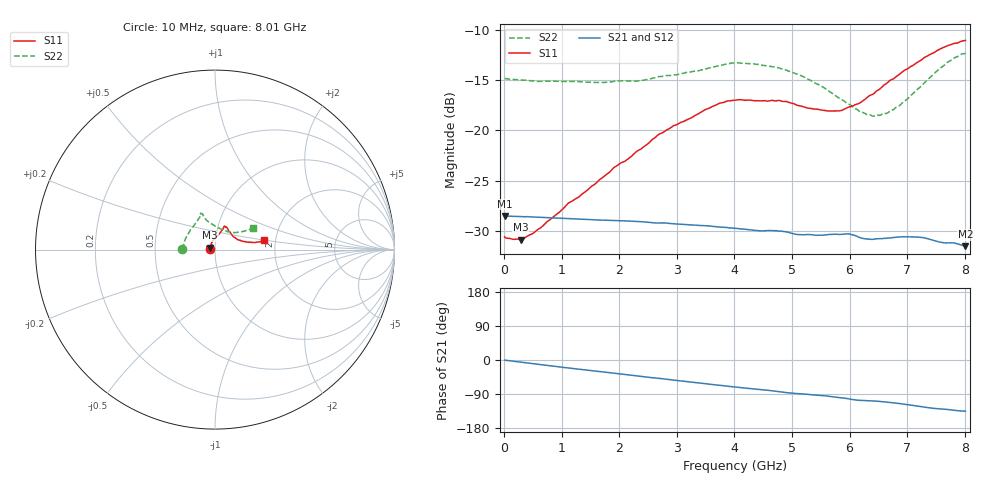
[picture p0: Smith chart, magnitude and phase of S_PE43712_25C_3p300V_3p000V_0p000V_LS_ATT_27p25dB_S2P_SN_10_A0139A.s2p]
! DEVICE ID: PE43712
! File Path: z:\PE43713\PE43713_CHAR_NOM_04292014\AMB\3p300\LS_ATT_27p25dB\PE43713_AMB_3p300V_3p000V_0p000V_LS_ATT_27p25dB_S2P_SN_10_A0139A.s2p
! Serial: 10
! Lot: A0139A
! Temp: 25C
! VDD: 3.300
! VSS: 0.000
! Control_Hi: 3.000
! Control_Lo: 0.000
! Attenuation Step: 27.25dB
! Port 1: RF1
! Port 2: RF2
! ThroughPath:1-2
! IDD: 0.0001454839
! ISS: -9.96e-008
#  Hz  S  RI  R  50
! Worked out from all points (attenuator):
!   801 points, 10 MHz to 8.01 GHz, reference 50 ohm
!   highest |S21| = -28.51 dB at 10 MHz (marker M1); lowest = -31.5 dB at 8.01 GHz (marker M2)
!   lowest |S11| = -30.9 dB at 290 MHz (marker M3), VSWR 1.06, Z = 47.4 + j1.03 ohm
!   |S11| at or under -10 dB: start of sweep to end of sweep
!   |S22| runs from -18.6 to -12.3 dB; largest |S21 - S12| = 0.00013
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1e7  -0.0296 0.000769  0.0375 -0.000171  0.0376 -0.000142  -0.1812 0.00116
2.9e8  -0.0265 0.0109  0.0372 -0.00374  0.0372 -0.00374  -0.1771 0.0185
6.4e8  -0.0235 0.0231  0.0361 -0.00792  0.0361 -0.00792  -0.171 0.0386
1.12e9  -0.018 0.0397  0.034 -0.0131  0.034 -0.0131  -0.1624 0.0655
1.35e9  -0.0133 0.0463  0.0328 -0.0154  0.0328 -0.0154  -0.1566 0.0764
2.31e9  0.0137 0.0777  0.0262 -0.0236  0.0262 -0.0236  -0.1225 0.1265
2.68e9  0.0266 0.0915  0.0231 -0.0259  0.0231 -0.0259  -0.1069 0.1509
3.5e9  0.0457 0.1186  0.0155 -0.0298  0.0155 -0.0298  -0.0838 0.184
3.74e9  0.0495 0.1271  0.0131 -0.0304  0.0131 -0.0304  -0.0815 0.1938
4.01e9  0.0533 0.131  0.0105 -0.0309  0.0105 -0.0309  -0.0806 0.201
4.76e9  0.0637 0.1256  0.0037 -0.0314  0.00372 -0.0314  -0.0666 0.1937
5.35e9  0.0803 0.0999  -0.00099 -0.0303  -0.00101 -0.0302  -0.0515 0.168
5.87e9  0.1047 0.0702  -0.00522 -0.03  -0.00521 -0.03  -0.0152 0.141
5.99e9  0.113 0.0657  -0.00678 -0.0298  -0.00672 -0.0298  -0.00443 0.1349
6.18e9  0.1249 0.0562  -0.00836 -0.0282  -0.0083 -0.0281  0.0148 0.1228
6.39e9  0.1417 0.0509  -0.00885 -0.0273  -0.00879 -0.0273  0.0383 0.1116
6.68e9  0.1698 0.0437  -0.0107 -0.0271  -0.0107 -0.0271  0.0735 0.0993
6.87e9  0.1862 0.0406  -0.0125 -0.0268  -0.0125 -0.0268  0.0928 0.0955
7.17e9  0.2139 0.0399  -0.0154 -0.0252  -0.0153 -0.0252  0.1269 0.0966
7.55e9  0.2484 0.0434  -0.0175 -0.0218  -0.0175 -0.0217  0.1714 0.1052
7.81e9  0.2659 0.0482  -0.0186 -0.0204  -0.0186 -0.0204  0.198 0.1142
8.01e9  0.275 0.0522  -0.0188 -0.0188  -0.0187 -0.0189  0.211 0.1178
